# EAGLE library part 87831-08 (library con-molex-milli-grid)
HEADER
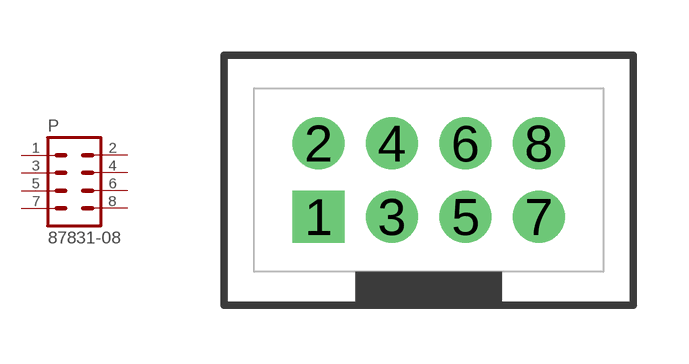
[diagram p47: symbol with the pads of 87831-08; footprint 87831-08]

Designator prefix P

## 87831-08  [87831-08]
1  1  pas
2  2  pas
3  3  pas
4  4  pas
5  5  pas
6  6  pas
7  7  pas
8  8  pas

## Footprint 87831-08 (pad centres in mm)
HEADER Dual Row, Shrouded, Vertical
drill 0.914 square: 1 -3,-1
drill 0.914: 2 -3,1; 3 -1,-1; 4 -1,1; 5 1,-1; 6 1,1; 7 3,-1; 8 3,1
